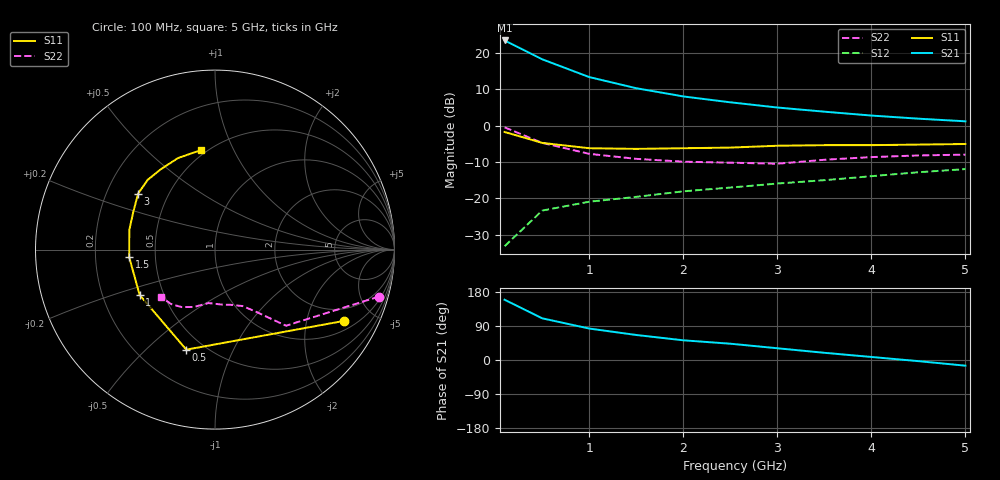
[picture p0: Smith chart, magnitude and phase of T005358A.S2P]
!AT-00535
!S-PARAMETERS at Vce=8V  Ic=5mA.  LAST UPDATED 07-21-92
# ghz s ma r 50
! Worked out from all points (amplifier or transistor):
!   11 points, 100 MHz to 5 GHz, reference 50 ohm
!   highest |S21| = 23.5 dB at 100 MHz (marker M1)
!   |S21| within 3 dB of that: start of sweep to 331.3 MHz
!   unconditionally stable (mu >= 1): 1.55 GHz to 4.82 GHz
!   at 500 MHz: K = 0.47, MSG = 20.8 dB, |S12| = -23.3 dB
!   at 2.5 GHz: K = 1.14, MAG = 9.5 dB, |S12| = -17.0 dB
!   at 5 GHz: K = 0.99, MSG = 6.6 dB, |S12| = -11.9 dB
!   S11 on the Smith chart (normalised r, x): 100 MHz: 1.38, -3.34; 500 MHz: 0.40, -0.67; 1 GHz: 0.37, -0.24; 1.5 GHz: 0.35, -0.04; 3 GHz: 0.34, +0.29; 5 GHz: 0.47, +0.75
0.1  0.82 -29.0  14.9 159.0  0.022 69.0  0.95 -16.0
0.5  0.58 -106.0  8.2 110.0  0.068 44.0  0.58 -47.0
1  0.49 -149.0  4.67 83.0  0.09 37.0  0.41 -57.0
1.5  0.48 -175.0  3.28 66.0  0.105 39.0  0.35 -64.0
2  0.49 167.0  2.53 52.0  0.125 37.0  0.32 -74.0
2.5  0.5 156.0  2.1 43.0  0.141 41.0  0.31 -82.0
3  0.53 144.0  1.78 31.0  0.16 39.0  0.3 -97.0
3.5  0.54 134.0  1.56 19.0  0.178 36.0  0.34 -110.0
4  0.54 124.0  1.38 8.0  0.202 34.0  0.37 -120.0
4.5  0.55 112.0  1.25 -3.0  0.229 29.0  0.39 -129.0
5  0.56 98.0  1.15 -15.0  0.253 23.0  0.4 -139.0
